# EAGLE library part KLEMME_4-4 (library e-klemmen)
Klemme 4 4
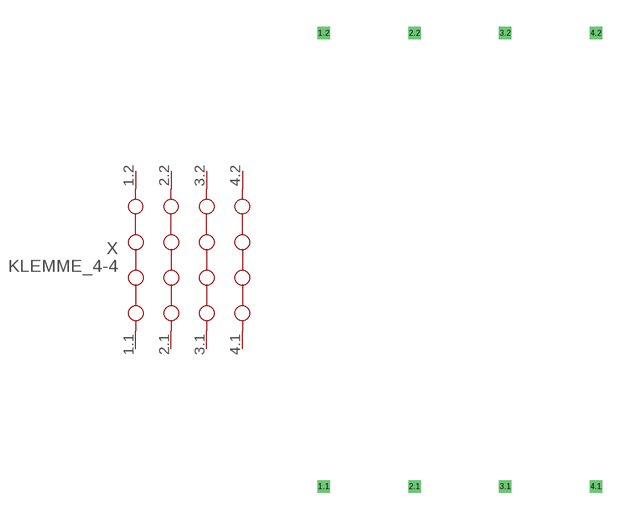
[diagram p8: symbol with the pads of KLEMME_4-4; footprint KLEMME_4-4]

Designator prefix X

## KLEMME_4-4  [KLEMME_4-4]
1.1  1.1  pas
1.2  1.2  pas
2.1  2.1  pas
2.2  2.2  pas
3.1  3.1  pas
3.2  3.2  pas
4.1  4.1  pas
4.2  4.2  pas

## Footprint KLEMME_4-4 (pad centres in mm)
Dummy
drill 0.2 pad 0.6 square: 1.1 0,-12.7; 1.2 0,12.7; 2.1 5.08,-12.7; 2.2 5.08,12.7; 3.1 10.16,-12.7; 3.2 10.16,12.7; 4.1 15.24,-12.7; 4.2 15.24,12.7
